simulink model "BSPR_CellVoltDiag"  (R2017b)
settings: Solver=FixedStepDiscrete  StartTime=0.0  StopTime=10.0  FixedStep=0.02  RelTol=1e-3  EnableMultiTasking=on
undefined symbols (not defined in the file): bin2dec, BSPR_bCellVoltAlrmDiag_C, BSPR_CellNplDetVoltThres_C, BSPR_cntCellAvlNum_C, BSPR_cntCellVltRngEnvtCsdr_CW, BSPR_cntCellVoltNplDiag_CW, BSPR_cntCellVoltRngDiag_CW, BSPR_cntModuAvlNum_C, BSPR_cntUCellNplErrThres_C, BSPR_cntUCellNplOkThres_C, BSPR_cntVoltCellMeanSwt_CW, BSPR_cofCurrFltCellRng_C, BSPR_iCellVoltRngCurrHi_C, BSPR_iCellVoltRngCurrLo_C, BSPR_iCurrHopFltDiff_C, BSPR_tBattTempCellVoltRngHi_C, BSPR_tBattTempCellVoltRngLo_C, BSPR_tEnvTCellVoltRngHi_C, BSPR_tEnvTCellVoltRnglo_C, BSPR_tiCellVoltAlrm_C, BSPR_tiCellVoltDiagTask_C, BSPR_tiCellVoltFault_C, BSPR_tiCellVoltFusf_C, BSPR_tiCellVoltWarn_C, BSPR_tiUCellNplErrThres_C, BSPR_tiUCellNplOkThres_C, BSPR_uCellVoltNplDiag_CUR, BSPR_uCellVoltNplDiag_CUR_X, BSPR_uCellVoltRng_CUR_X, BSPR_uCellVoltRng_CUR_Y, BSPR_uCellVoltRngHiFault_CUR, BSPR_uCellVoltRngHiFusf_CUR, BSPR_uCellVoltRngHiWarnAlrm_CUR, BSPR_uCellVoltRngLoFault_CUR, BSPR_uCellVoltRngLoFusf_CUR, BSPR_uCellVoltRngLoWarnAlrm_CUR
libraries: simulink x68, AIWAYS_Powertrain_BMS_lib x9
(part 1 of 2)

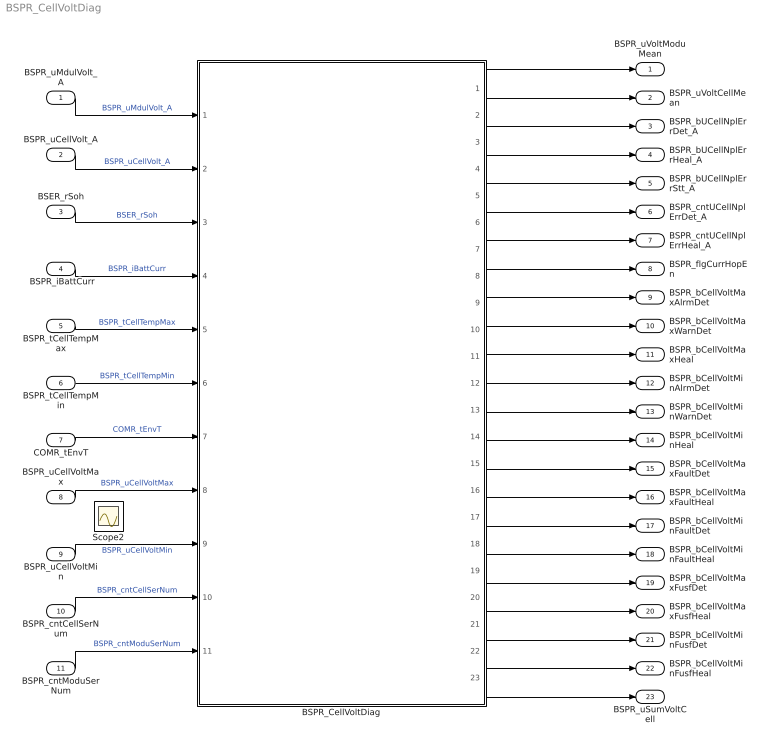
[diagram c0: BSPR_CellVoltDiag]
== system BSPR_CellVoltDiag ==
  BSPR_uMdulVolt_A : Inport
  BSPR_uCellVolt_A : Inport  Port=2
  BSER_rSoh : Inport  Port=3
  " BSPR_iBattCurr" : Inport  Port=4
  BSPR_tCellTempMax : Inport  Port=5
  BSPR_tCellTempMin : Inport  Port=6
  COMR_tEnvT : Inport  Port=7
  BSPR_uCellVoltMax : Inport  Port=8
  BSPR_uCellVoltMin : Inport  Port=9
  BSPR_cntCellSerNum : Inport  Port=10
  BSPR_cntModuSerNum : Inport  Port=11
  BSPR_CellVoltDiag : Subsystem
  BSPR_uVoltModuMean : Outport
  BSPR_uVoltCellMean : Outport  Port=2
  BSPR_bUCellNplErrDet_A : Outport  Port=3
  BSPR_bUCellNplErrHeal_A : Outport  Port=4
  BSPR_bUCellNplErrStt_A : Outport  Port=5
  BSPR_cntUCellNplErrDet_A : Outport  Port=6
  BSPR_cntUCellNplErrHeal_A : Outport  Port=7
  BSPR_flgCurrHopEn : Outport  Port=8
  BSPR_bCellVoltMaxAlrmDet : Outport  Port=9
  BSPR_bCellVoltMaxWarnDet : Outport  Port=10
  BSPR_bCellVoltMaxHeal : Outport  Port=11
  BSPR_bCellVoltMinAlrmDet : Outport  Port=12
  BSPR_bCellVoltMinWarnDet : Outport  Port=13
  BSPR_bCellVoltMinHeal : Outport  Port=14
  BSPR_bCellVoltMaxFaultDet : Outport  Port=15
  BSPR_bCellVoltMaxFaultHeal : Outport  Port=16
  BSPR_bCellVoltMinFaultDet : Outport  Port=17
  BSPR_bCellVoltMinFaultHeal : Outport  Port=18
  BSPR_bCellVoltMaxFusfDet : Outport  Port=19
  BSPR_bCellVoltMaxFusfHeal : Outport  Port=20
  BSPR_bCellVoltMinFusfDet : Outport  Port=21
  BSPR_bCellVoltMinFusfHeal : Outport  Port=22
  BSPR_uSumVoltCell : Outport  Port=23
  Scope2 : Scope
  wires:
  BSPR_uMdulVolt_A/1 -> BSPR_CellVoltDiag/1(BSPR_uMdulVolt_A)  "BSPR_uMdulVolt_A"
  BSPR_uCellVolt_A/1 -> BSPR_CellVoltDiag/2(BSPR_uCellVolt_A)  "BSPR_uCellVolt_A"
  BSER_rSoh/1 -> BSPR_CellVoltDiag/3(BSER_rSoh)  "BSER_rSoh"
  " BSPR_iBattCurr"/1 -> BSPR_CellVoltDiag/4(BSPR_iBattCurr)  "BSPR_iBattCurr"
  BSPR_tCellTempMax/1 -> BSPR_CellVoltDiag/5(BSPR_tCellTempMax)  "BSPR_tCellTempMax"
  BSPR_tCellTempMin/1 -> BSPR_CellVoltDiag/6(BSPR_tCellTempMin)  "BSPR_tCellTempMin"
  COMR_tEnvT/1 -> BSPR_CellVoltDiag/7(COMR_tEnvT)  "COMR_tEnvT"
  BSPR_uCellVoltMax/1 -> BSPR_CellVoltDiag/8(BSPR_uCellVoltMax)  "BSPR_uCellVoltMax"
  BSPR_uCellVoltMin/1 -> BSPR_CellVoltDiag/9(BSPR_uCellVoltMin)  "BSPR_uCellVoltMin"
  BSPR_CellVoltDiag/1(BSPR_uVoltModuMean) -> BSPR_uVoltModuMean/1
  BSPR_CellVoltDiag/2(BSPR_uVoltCellMean) -> BSPR_uVoltCellMean/1
  BSPR_CellVoltDiag/3(BSPR_bUCellNplErrDet_A) -> BSPR_bUCellNplErrDet_A/1
  BSPR_CellVoltDiag/4(BSPR_bUCellNplErrHeal_A) -> BSPR_bUCellNplErrHeal_A/1
  BSPR_CellVoltDiag/5(BSPR_bUCellNplErrStt_A) -> BSPR_bUCellNplErrStt_A/1
  BSPR_CellVoltDiag/6(BSPR_cntUCellNplErrDet_A) -> BSPR_cntUCellNplErrDet_A/1
  BSPR_CellVoltDiag/7(BSPR_cntUCellNplErrHeal_A) -> BSPR_cntUCellNplErrHeal_A/1
  BSPR_CellVoltDiag/8(BSPR_flgCurrHopEn) -> BSPR_flgCurrHopEn/1
  BSPR_CellVoltDiag/9(BSPR_bCellVoltMaxAlrmDet) -> BSPR_bCellVoltMaxAlrmDet/1
  BSPR_CellVoltDiag/10(BSPR_bCellVoltMaxWarnDet) -> BSPR_bCellVoltMaxWarnDet/1
  BSPR_CellVoltDiag/11(BSPR_bCellVoltMaxHeal) -> BSPR_bCellVoltMaxHeal/1
  BSPR_CellVoltDiag/12(BSPR_bCellVoltMinAlrmDet) -> BSPR_bCellVoltMinAlrmDet/1
  BSPR_CellVoltDiag/13(BSPR_bCellVoltMinWarnDet) -> BSPR_bCellVoltMinWarnDet/1
  BSPR_CellVoltDiag/14(BSPR_bCellVoltMinHeal) -> BSPR_bCellVoltMinHeal/1
  BSPR_CellVoltDiag/15(BSPR_bCellVoltMaxFaultDet) -> BSPR_bCellVoltMaxFaultDet/1
  BSPR_CellVoltDiag/16(BSPR_bCellVoltMaxFaultHeal) -> BSPR_bCellVoltMaxFaultHeal/1
  BSPR_CellVoltDiag/17(BSPR_bCellVoltMinFaultDet) -> BSPR_bCellVoltMinFaultDet/1
  BSPR_CellVoltDiag/18(BSPR_bCellVoltMinFaultHeal) -> BSPR_bCellVoltMinFaultHeal/1
  BSPR_CellVoltDiag/19(BSPR_bCellVoltMaxFusfDet) -> BSPR_bCellVoltMaxFusfDet/1
  BSPR_CellVoltDiag/20(BSPR_bCellVoltMaxFusfHeal) -> BSPR_bCellVoltMaxFusfHeal/1
  BSPR_CellVoltDiag/21(BSPR_bCellVoltMinFusfDet) -> BSPR_bCellVoltMinFusfDet/1
  BSPR_CellVoltDiag/22(BSPR_bCellVoltMinFusfHeal) -> BSPR_bCellVoltMinFusfHeal/1
  BSPR_cntCellSerNum/1 -> BSPR_CellVoltDiag/10(BSPR_cntCellSerNum)  "BSPR_cntCellSerNum"
  BSPR_CellVoltDiag/23(BSPR_uSumVoltCell) -> BSPR_uSumVoltCell/1
  BSPR_cntModuSerNum/1 -> BSPR_CellVoltDiag/11(BSPR_cntModuSerNum)  "BSPR_cntModuSerNum"

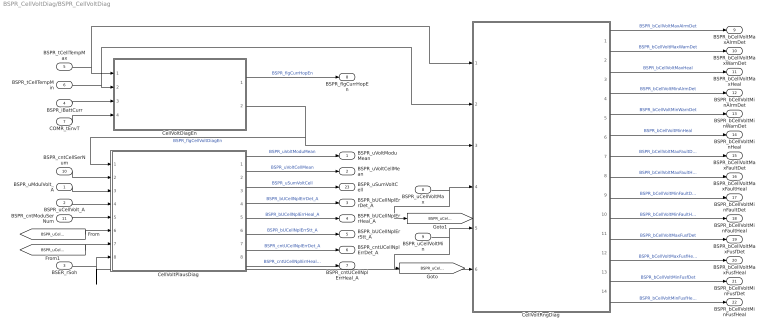
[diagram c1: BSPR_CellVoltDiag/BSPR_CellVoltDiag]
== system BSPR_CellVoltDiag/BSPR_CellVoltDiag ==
  BSPR_uMdulVolt_A : Inport
  BSPR_uCellVolt_A : Inport  Port=2
  BSER_rSoh : Inport  Port=3
  BSPR_iBattCurr : Inport  Port=4
  BSPR_tCellTempMax : Inport  Port=5
  BSPR_tCellTempMin : Inport  Port=6
  COMR_tEnvT : Inport  Port=7
  BSPR_uCellVoltMax : Inport  Port=8
  BSPR_uCellVoltMin : Inport  Port=9
  BSPR_cntCellSerNum : Inport  Port=10
  BSPR_cntModuSerNum : Inport  Port=11
  CellVoltDiagEn : Subsystem
  CellVoltPlausDiag : Subsystem
  CellVoltRngDiag : Subsystem
  BSPR_uVoltModuMean : Outport
  BSPR_uVoltCellMean : Outport  Port=2
  BSPR_bUCellNplErrDet_A : Outport  Port=3
  BSPR_bUCellNplErrHeal_A : Outport  Port=4
  BSPR_bUCellNplErrStt_A : Outport  Port=5
  BSPR_cntUCellNplErrDet_A : Outport  Port=6
  BSPR_cntUCellNplErrHeal_A : Outport  Port=7
  BSPR_flgCurrHopEn : Outport  Port=8
  BSPR_bCellVoltMaxAlrmDet : Outport  Port=9
  BSPR_bCellVoltMaxWarnDet : Outport  Port=10
  BSPR_bCellVoltMaxHeal : Outport  Port=11
  BSPR_bCellVoltMinAlrmDet : Outport  Port=12
  BSPR_bCellVoltMinWarnDet : Outport  Port=13
  BSPR_bCellVoltMinHeal : Outport  Port=14
  BSPR_bCellVoltMaxFaultDet : Outport  Port=15
  BSPR_bCellVoltMaxFaultHeal : Outport  Port=16
  BSPR_bCellVoltMinFaultDet : Outport  Port=17
  BSPR_bCellVoltMinFaultHeal : Outport  Port=18
  BSPR_bCellVoltMaxFusfDet : Outport  Port=19
  BSPR_bCellVoltMaxFusfHeal : Outport  Port=20
  BSPR_bCellVoltMinFusfDet : Outport  Port=21
  BSPR_bCellVoltMinFusfHeal : Outport  Port=22
  BSPR_uSumVoltCell : Outport  Port=23
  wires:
  BSPR_uCellVolt_A/1 -> CellVoltPlausDiag/4(BSPR_uCellVolt_A)
  BSPR_uMdulVolt_A/1 -> CellVoltPlausDiag/3(BSPR_uMdulVolt_A)
  BSER_rSoh/1 -> CellVoltPlausDiag/8(BSER_rSoh), CellVoltRngDiag/6(BSER_rSoh)
  CellVoltPlausDiag/1(BSPR_uVoltModuMean) -> BSPR_uVoltModuMean/1  "BSPR_uVoltModuMean"
  CellVoltPlausDiag/5(BSPR_bUCellNplErrHeal_A) -> BSPR_bUCellNplErrHeal_A/1  "BSPR_bUCellNplErrHeal_A"
  CellVoltPlausDiag/4(BSPR_bUCellNplErrDet_A) -> BSPR_bUCellNplErrDet_A/1  "BSPR_bUCellNplErrDet_A"
  CellVoltPlausDiag/2(BSPR_uVoltCellMean) -> BSPR_uVoltCellMean/1  "BSPR_uVoltCellMean"
  CellVoltPlausDiag/6(BSPR_bUCellNplErrStt_A) -> BSPR_bUCellNplErrStt_A/1  "BSPR_bUCellNplErrStt_A"
  CellVoltPlausDiag/7(BSPR_cntUCellNplErrDet_A) -> BSPR_cntUCellNplErrDet_A/1  "BSPR_cntUCellNplErrDet_A"
  CellVoltPlausDiag/8(BSPR_cntUCellNplErrHeal_A) -> BSPR_cntUCellNplErrHeal_A/1  "BSPR_cntUCellNplErrHeal_A"
  CellVoltDiagEn/1(BSPR_flgCurrHopEn) -> BSPR_flgCurrHopEn/1  "BSPR_flgCurrHopEn"
  BSPR_tCellTempMax/1 -> CellVoltDiagEn/1(BSPR_tCellTempMax), CellVoltRngDiag/1(BSPR_tCellTempMax)
  BSPR_tCellTempMin/1 -> CellVoltRngDiag/2(BSPR_tCellTempMin), CellVoltDiagEn/2(BSPR_tCellTempMin)
  BSPR_iBattCurr/1 -> CellVoltDiagEn/3(BSPR_iBattCurr)
  COMR_tEnvT/1 -> CellVoltDiagEn/4(COMR_tEnvT)
  CellVoltDiagEn/2(BSPR_flgCellVoltDiagEn) -> CellVoltPlausDiag/1(BSPR_flgCellVoltDiagEn), CellVoltRngDiag/3(BSPR_flgCellVoltDiagEn)  "BSPR_flgCellVoltDiagEn"
  CellVoltRngDiag/1(BSPR_bCellVoltMaxAlrmDet) -> BSPR_bCellVoltMaxAlrmDet/1  "BSPR_bCellVoltMaxAlrmDet"
  CellVoltRngDiag/2(BSPR_bCellVoltMaxWarnDet) -> BSPR_bCellVoltMaxWarnDet/1  "BSPR_bCellVoltMaxWarnDet"
  CellVoltRngDiag/3(BSPR_bCellVoltMaxHeal) -> BSPR_bCellVoltMaxHeal/1  "BSPR_bCellVoltMaxHeal"
  CellVoltRngDiag/4(BSPR_bCellVoltMinAlrmDet) -> BSPR_bCellVoltMinAlrmDet/1  "BSPR_bCellVoltMinAlrmDet"
  CellVoltRngDiag/5(BSPR_bCellVoltMinWarnDet) -> BSPR_bCellVoltMinWarnDet/1  "BSPR_bCellVoltMinWarnDet"
  CellVoltRngDiag/7(BSPR_bCellVoltMaxFaultDet) -> BSPR_bCellVoltMaxFaultDet/1  "BSPR_bCellVoltMaxFaultDet"
  CellVoltRngDiag/9(BSPR_bCellVoltMinFaultDet) -> BSPR_bCellVoltMinFaultDet/1  "BSPR_bCellVoltMinFaultDet"
  CellVoltRngDiag/10(BSPR_bCellVoltMinFaultHeal) -> BSPR_bCellVoltMinFaultHeal/1  "BSPR_bCellVoltMinFaultHeal"
  CellVoltRngDiag/11(BSPR_bCellVoltMaxFusfDet) -> BSPR_bCellVoltMaxFusfDet/1  "BSPR_bCellVoltMaxFusfDet"
  CellVoltRngDiag/13(BSPR_bCellVoltMinFusfDet) -> BSPR_bCellVoltMinFusfDet/1  "BSPR_bCellVoltMinFusfDet"
  CellVoltRngDiag/14(BSPR_bCellVoltMinFusfHeal) -> BSPR_bCellVoltMinFusfHeal/1  "BSPR_bCellVoltMinFusfHeal"
  BSPR_uCellVoltMax/1 -> [BSPR_uCellVoltMax], CellVoltRngDiag/4(BSPR_uCellVoltMax)
  BSPR_uCellVoltMin/1 -> [BSPR_uCellVoltMin], CellVoltRngDiag/5(BSPR_uCellVoltMin)
  CellVoltRngDiag/6(BSPR_bCellVoltMinHeal) -> BSPR_bCellVoltMinHeal/1  "BSPR_bCellVoltMinHeal"
  CellVoltRngDiag/8(BSPR_bCellVoltMaxFaultHeal) -> BSPR_bCellVoltMaxFaultHeal/1  "BSPR_bCellVoltMaxFaultHeal"
  CellVoltRngDiag/12(BSPR_bCellVoltMaxFusfHeal) -> BSPR_bCellVoltMaxFusfHeal/1  "BSPR_bCellVoltMaxFusfHeal"
  BSPR_cntCellSerNum/1 -> CellVoltPlausDiag/2(BSPR_cntCellSerNum)
  CellVoltPlausDiag/3(BSPR_uSumVoltCell) -> BSPR_uSumVoltCell/1  "BSPR_uSumVoltCell"
  BSPR_cntModuSerNum/1 -> CellVoltPlausDiag/5(BSPR_cntModuSerNum)
  [BSPR_uCellVoltMin] -> CellVoltPlausDiag/6(BSPR_uCellVoltMin)
  [BSPR_uCellVoltMax] -> CellVoltPlausDiag/7(BSPR_uCellVoltMax)

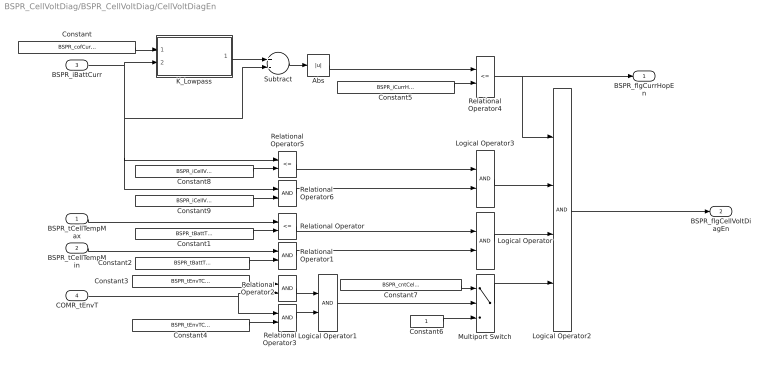
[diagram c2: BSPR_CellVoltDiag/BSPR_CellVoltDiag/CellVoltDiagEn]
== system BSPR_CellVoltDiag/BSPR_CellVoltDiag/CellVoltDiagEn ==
  BSPR_tCellTempMax : Inport
  BSPR_tCellTempMin : Inport  Port=2
  BSPR_iBattCurr : Inport  Port=3
  COMR_tEnvT : Inport  Port=4
  Abs : Abs
  Constant : Constant  Value=BSPR_cofCurrFltCellRng_C
  Constant1 : Constant  Value=BSPR_tBattTempCellVoltRngHi_C
  Constant2 : Constant  Value=BSPR_tBattTempCellVoltRngLo_C
  Constant3 : Constant  Value=BSPR_tEnvTCellVoltRngHi_C
  Constant4 : Constant  Value=BSPR_tEnvTCellVoltRnglo_C
  Constant5 : Constant  Value=BSPR_iCurrHopFltDiff_C
  Constant6 : Constant
  Constant7 : Constant  Value=BSPR_cntCellVltRngEnvtCsdr_CW  OutMin=[0]  OutMax=[1]
  Constant8 : Constant  Value=BSPR_iCellVoltRngCurrHi_C
  Constant9 : Constant  Value=BSPR_iCellVoltRngCurrLo_C
  K_Lowpass : Subsystem  TreatAsAtomicUnit=on  RTWFcnName=K_Lowpass  RTWFileName=SrvLib
  Logical Operator : Logic  AllPortsSameDT=off  OutDataTypeStr=boolean
  Logical Operator1 : Logic  AllPortsSameDT=off  OutDataTypeStr=boolean
  Logical Operator2 : Logic  Inputs=4  AllPortsSameDT=off  OutDataTypeStr=boolean
  Logical Operator3 : Logic  AllPortsSameDT=off  OutDataTypeStr=boolean
  Multiport Switch : MultiPortSwitch  DataPortOrder=Zero-based contiguous  Inputs=2
  Relational Operator : RelationalOperator  Operator=<=  OutDataTypeStr=boolean  RndMeth=Simplest
  Relational Operator{1..3,6} (4 alike) : RelationalOperator  OutDataTypeStr=boolean  RndMeth=Simplest
  Relational Operator4 : RelationalOperator  Operator=<=  OutDataTypeStr=boolean  RndMeth=Simplest
  Relational Operator5 : RelationalOperator  Operator=<=  OutDataTypeStr=boolean  RndMeth=Simplest
  Subtract : Sum  Inputs=+-
  BSPR_flgCurrHopEn : Outport
  BSPR_flgCellVoltDiagEn : Outport  Port=2
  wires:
  K_Lowpass/1(y) -> Subtract/1
  Subtract/1 -> Abs/1
  Abs/1 -> Relational Operator4/1
  Constant6/1 -> Multiport Switch/3
  Multiport Switch/1 -> Logical Operator2/4
  Constant3/1 -> Relational Operator2/1
  Constant4/1 -> Relational Operator3/2
  COMR_tEnvT/1 -> Relational Operator3/1, Relational Operator2/2
  Constant1/1 -> Relational Operator/2
  Constant2/1 -> Relational Operator1/2
  BSPR_tCellTempMin/1 -> Relational Operator1/1
  BSPR_iBattCurr/1 -> K_Lowpass/2(u), Relational Operator6/1, Relational Operator5/1, Subtract/2
  BSPR_tCellTempMax/1 -> Relational Operator/1
  Relational Operator1/1 -> Logical Operator/2
  Relational Operator3/1 -> Logical Operator1/2
  Relational Operator2/1 -> Logical Operator1/1
  Constant7/1 -> Multiport Switch/1
  Relational Operator/1 -> Logical Operator/1
  Logical Operator1/1 -> Multiport Switch/2
  Relational Operator4/1 -> BSPR_flgCurrHopEn/1, Logical Operator2/1
  Constant5/1 -> Relational Operator4/2
  Logical Operator/1 -> Logical Operator2/3
  Logical Operator2/1 -> BSPR_flgCellVoltDiagEn/1
  Constant/1 -> K_Lowpass/1(k)
  Constant9/1 -> Relational Operator6/2
  Constant8/1 -> Relational Operator5/2
  Relational Operator5/1 -> Logical Operator3/1
  Relational Operator6/1 -> Logical Operator3/2
  Logical Operator3/1 -> Logical Operator2/2

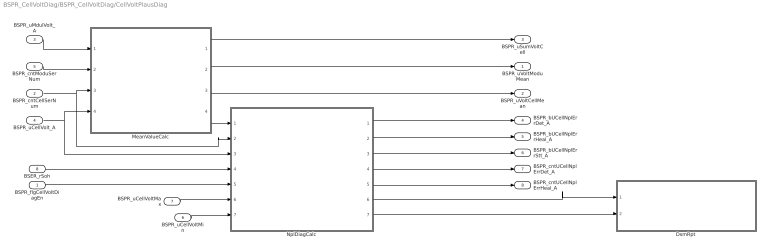
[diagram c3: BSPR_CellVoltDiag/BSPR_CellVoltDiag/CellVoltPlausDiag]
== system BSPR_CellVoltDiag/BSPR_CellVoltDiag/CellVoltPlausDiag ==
  BSPR_flgCellVoltDiagEn : Inport
  BSPR_cntCellSerNum : Inport  Port=2
  BSPR_uMdulVolt_A : Inport  Port=3
  BSPR_uCellVolt_A : Inport  Port=4
  BSPR_cntModuSerNum : Inport  Port=5
  BSPR_uCellVoltMin : Inport  Port=6
  BSPR_uCellVoltMax : Inport  Port=7
  BSER_rSoh : Inport  Port=8
  DsmRpt : Subsystem
  MeanValueCalc : Subsystem
  NplDiagCalc : Subsystem
  BSPR_uVoltModuMean : Outport
  BSPR_uVoltCellMean : Outport  Port=2
  BSPR_uSumVoltCell : Outport  Port=3
  BSPR_bUCellNplErrDet_A : Outport  Port=4  InitialOutput=[0]
  BSPR_bUCellNplErrHeal_A : Outport  Port=5  InitialOutput=[0]
  BSPR_bUCellNplErrStt_A : Outport  Port=6  InitialOutput=[0]
  BSPR_cntUCellNplErrDet_A : Outport  Port=7  InitialOutput=[0]
  BSPR_cntUCellNplErrHeal_A : Outport  Port=8  InitialOutput=[0]
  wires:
  BSPR_uMdulVolt_A/1 -> MeanValueCalc/1(BSPR_uMdulVolt_A)
  MeanValueCalc/2(BSPR_uVoltModuMean) -> BSPR_uVoltModuMean/1
  MeanValueCalc/4(BSPR_uCellVoltMeanCoord) -> NplDiagCalc/1(BSPR_uCellVoltMeanCoord)
  NplDiagCalc/2(BSPR_bUCellNplErrHeal_A) -> BSPR_bUCellNplErrHeal_A/1
  NplDiagCalc/1(BSPR_bUCellNplErrDet_A) -> BSPR_bUCellNplErrDet_A/1
  BSER_rSoh/1 -> NplDiagCalc/4(BSER_rSoh)
  MeanValueCalc/3(BSPR_uVoltCellMean) -> BSPR_uVoltCellMean/1
  NplDiagCalc/3(BSPR_bUCellNplErrStt_A) -> BSPR_bUCellNplErrStt_A/1
  NplDiagCalc/4(BSPR_cntUCellNplErrDet_A) -> BSPR_cntUCellNplErrDet_A/1
  NplDiagCalc/5(BSPR_cntUCellNplErrHeal_A) -> BSPR_cntUCellNplErrHeal_A/1
  BSPR_uCellVolt_A/1 -> MeanValueCalc/4(BSPR_uCellVolt_A), NplDiagCalc/3(BSPR_uCellVolt_A)
  BSPR_flgCellVoltDiagEn/1 -> NplDiagCalc/5(BSPR_flgCellVoltDiagEn)
  MeanValueCalc/1(BSPR_uSumVoltCell) -> BSPR_uSumVoltCell/1
  BSPR_cntCellSerNum/1 -> MeanValueCalc/3(BSPR_cntCellSerNum), NplDiagCalc/2(BSPR_cntCellSerNum)
  BSPR_cntModuSerNum/1 -> MeanValueCalc/2(BSPR_cntModuSerNum)
  BSPR_uCellVoltMin/1 -> NplDiagCalc/7(BSPR_uCellVoltMin)
  BSPR_uCellVoltMax/1 -> NplDiagCalc/6(BSPR_uCellVoltMax)
  NplDiagCalc/6(BSPR_bUCellNplErrDet_flg) -> DsmRpt/1(BSPR_bUCellNplErrDet_flg)
  NplDiagCalc/7(BSPR_bUCellNplErrHeal_flg) -> DsmRpt/2(BSPR_bUCellNplErrHeal_flg)

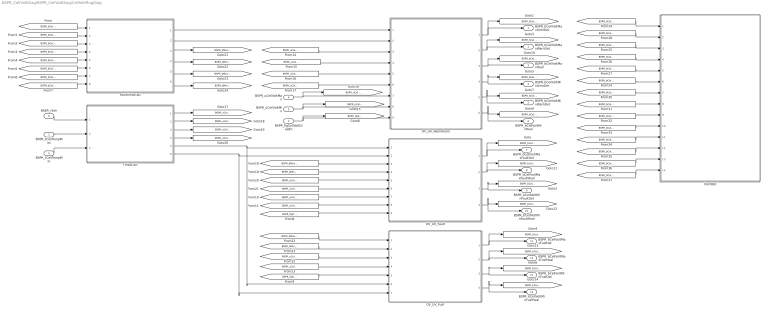
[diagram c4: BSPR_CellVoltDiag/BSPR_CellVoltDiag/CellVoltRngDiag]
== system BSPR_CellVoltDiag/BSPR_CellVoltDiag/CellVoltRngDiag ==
  BSPR_tCellTempMax : Inport
  BSPR_tCellTempMin : Inport  Port=2
  BSPR_flgCellVoltDiagEn : Inport  Port=3
  BSPR_uCellVoltMax : Inport  Port=4
  BSPR_uCellVoltMin : Inport  Port=5
  BSER_rSoh : Inport  Port=6
  DsmRpt : Subsystem
  FaultInhibCalc : Subsystem
  OV_UV_Fault : Subsystem
  OV_UV_Fusf : Subsystem
  OV_UV_WarnAlarm : Subsystem
  ThresCalc : Subsystem
  BSPR_bCellVoltMaxAlrmDet : Outport  InitialOutput=[0]
  BSPR_bCellVoltMaxWarnDet : Outport  Port=2  InitialOutput=[0]
  BSPR_bCellVoltMaxHeal : Outport  Port=3  InitialOutput=[0]
  BSPR_bCellVoltMinAlrmDet : Outport  Port=4  InitialOutput=[0]
  BSPR_bCellVoltMinWarnDet : Outport  Port=5  InitialOutput=[0]
  BSPR_bCellVoltMinHeal : Outport  Port=6  InitialOutput=[0]
  BSPR_bCellVoltMaxFaultDet : Outport  Port=7  InitialOutput=[0]
  BSPR_bCellVoltMaxFaultHeal : Outport  Port=8  InitialOutput=[0]
  BSPR_bCellVoltMinFaultDet : Outport  Port=9  InitialOutput=[0]
  BSPR_bCellVoltMinFaultHeal : Outport  Port=10  InitialOutput=[0]
  BSPR_bCellVoltMaxFusfDet : Outport  Port=11  InitialOutput=[0]
  BSPR_bCellVoltMaxFusfHeal : Outport  Port=12  InitialOutput=[0]
  BSPR_bCellVoltMinFusfDet : Outport  Port=13  InitialOutput=[0]
  BSPR_bCellVoltMinFusfHeal : Outport  Port=14  InitialOutput=[0]
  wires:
  OV_UV_WarnAlarm/6(BSPR_bCellVoltMinHeal) -> BSPR_bCellVoltMinHeal/1, [BSPR_bCellVoltMinHeal]
  OV_UV_WarnAlarm/5(BSPR_bCellVoltMinWarnDet) -> BSPR_bCellVoltMinWarnDet/1, [BSPR_bCellVoltMinWarnDet]
  OV_UV_WarnAlarm/4(BSPR_bCellVoltMinAlrmDet) -> BSPR_bCellVoltMinAlrmDet/1, [BSPR_bCellVoltMinAlrmDet]
  OV_UV_WarnAlarm/3(BSPR_bCellVoltMaxHeal) -> BSPR_bCellVoltMaxHeal/1, [BSPR_bCellVoltMaxHeal]
  OV_UV_WarnAlarm/2(BSPR_bCellVoltMaxWarnDet) -> BSPR_bCellVoltMaxWarnDet/1, [BSPR_bCellVoltMaxWarnDet]
  OV_UV_WarnAlarm/1(BSPR_bCellVoltMaxAlrmDet) -> BSPR_bCellVoltMaxAlrmDet/1, [BSPR_bCellVoltMaxAlrmDet]
  BSER_rSoh/1 -> ThresCalc/1(BSER_rSoh)
  OV_UV_Fault/1(BSPR_bCellVoltMaxFaultDet) -> [BSPR_bCellVoltMaxFaultDet], BSPR_bCellVoltMaxFaultDet/1
  OV_UV_Fault/3(BSPR_bCellVoltMinFaultDet) -> [BSPR_bCellVoltMinFaultDet], BSPR_bCellVoltMinFaultDet/1
  OV_UV_Fault/4(BSPR_bCellVoltMinFaultHeal) -> [BSPR_bCellVoltMinFaultHeal], BSPR_bCellVoltMinFaultHeal/1
  ThresCalc/5(BSPR_uCellVoltRngHiFusf) -> OV_UV_Fault/1(BSPR_uCellVoltRngHiFusf), OV_UV_Fusf/6(BSPR_uCellVoltRngHiFusf)
  ThresCalc/6(BSPR_uCellVoltRngLoFusf) -> OV_UV_Fault/2(BSPR_uCellVoltRngLoFusf), OV_UV_Fusf/7(BSPR_uCellVoltRngLoFusf)
  BSPR_uCellVoltMax/1 -> [BSPR_uCellVoltMax], OV_UV_WarnAlarm/7(BSPR_uCellVoltMax)
  BSPR_uCellVoltMin/1 -> [BSPR_uCellVoltMin], OV_UV_WarnAlarm/8(BSPR_uCellVoltMin)
  OV_UV_Fusf/1(BSPR_bCellVoltMaxFusfDet) -> BSPR_bCellVoltMaxFusfDet/1, [BSPR_bCellVoltMaxFusfDet]
  OV_UV_Fusf/2(BSPR_bCellVoltMaxFusfHeal) -> [BSPR_bCellVoltMaxFusfHeal], BSPR_bCellVoltMaxFusfHeal/1
  OV_UV_Fusf/3(BSPR_bCellVoltMinFusfDet) -> [BSPR_bCellVoltMinFusfDet], BSPR_bCellVoltMinFusfDet/1
  OV_UV_Fusf/4(BSPR_bCellVoltMinFusfHeal) -> [BSPR_bCellVoltMinFusfHeal], BSPR_bCellVoltMinFusfHeal/1
  [BSPR_bCellVoltMaxAlrmDet] -> FaultInhibCalc/1(BSPR_bCellVoltMaxAlrmDet)
  [BSPR_bCellVoltMaxWarnDet] -> FaultInhibCalc/2(BSPR_bCellVoltMaxWarnDet)
  [BSPR_bCellVoltMinAlrmDet] -> FaultInhibCalc/3(BSPR_bCellVoltMinAlrmDet)
  [BSPR_bCellVoltMinWarnDet] -> FaultInhibCalc/4(BSPR_bCellVoltMinWarnDet)
  [BSPR_bCellVoltMinFusfDet] -> FaultInhibCalc/8(BSPR_bCellVoltMinFusfDet)
  [BSPR_bCellVoltMaxFaultDet] -> FaultInhibCalc/5(BSPR_bCellVoltMaxFaultDet)
  [BSPR_bCellVoltMinFaultDet] -> FaultInhibCalc/6(BSPR_bCellVoltMinFaultDet)
  [BSPR_bCellVoltMaxFusfDet] -> FaultInhibCalc/7(BSPR_bCellVoltMaxFusfDet)
  FaultInhibCalc/1(BSPR_bMaxAlrmWarnInhib) -> OV_UV_WarnAlarm/1(BSPR_bMaxAlrmWarnInhib)
  FaultInhibCalc/2(BSPR_bMinAlrmWarnInhib) -> OV_UV_WarnAlarm/2(BSPR_bMinAlrmWarnInhib)
  BSPR_tCellTempMin/1 -> ThresCalc/3(BSPR_tCellTempMin)
  BSPR_tCellTempMax/1 -> ThresCalc/2(BSPR_tCellTempMax)
  BSPR_flgCellVoltDiagEn/1 -> OV_UV_WarnAlarm/9(BSPR_flgCellVoltDiagEn), [BSPR_flgCellVoltDiagEn]
  [BSPR_flgCellVoltDiagEn] -> OV_UV_Fault/9(BSPR_flgCellVoltDiagEn)
  [BSPR_flgCellVoltDiagEn] -> OV_UV_Fusf/5(BSPR_flgCellVoltDiagEn)
  OV_UV_Fault/2(BSPR_bCellVoltMaxFaultHeal) -> [BSPR_bCellVoltMaxFaultHeal], BSPR_bCellVoltMaxFaultHeal/1
  [BSPR_uCellVoltMin] -> OV_UV_Fault/8(BSPR_uCellVoltMin)
  [BSPR_uCellVoltMax] -> OV_UV_Fault/7(BSPR_uCellVoltMax)
  [BSPR_uCellVoltMax] -> OV_UV_Fusf/3(BSPR_uCellVoltMax)
  [BSPR_uCellVoltMin] -> OV_UV_Fusf/4(BSPR_uCellVoltMin)
  ThresCalc/1(BSPR_uCellVoltRngHiWarnAlrm) -> [BSPR_uCellVoltRngHiWarnAlrm]
  ThresCalc/2(BSPR_uCellVoltRngLoWarnAlrm) -> [BSPR_uCellVoltRngLoWarnAlrm]
  ThresCalc/3(BSPR_uCellVoltRngHiFault) -> [BSPR_uCellVoltRngHiFault]
  ThresCalc/4(BSPR_uCellVoltRngLoFault) -> [BSPR_uCellVoltRngLoFault]
  [BSPR_uCellVoltRngHiWarnAlrm] -> OV_UV_WarnAlarm/3(BSPR_uCellVoltRngHiWarnAlrm)
  [BSPR_uCellVoltRngLoWarnAlrm] -> OV_UV_WarnAlarm/4(BSPR_uCellVoltRngLoWarnAlrm)
  [BSPR_uCellVoltRngHiFault] -> OV_UV_WarnAlarm/5(BSPR_uCellVoltRngHiFault)
  [BSPR_uCellVoltRngLoFault] -> OV_UV_WarnAlarm/6(BSPR_uCellVoltRngLoFault)
  FaultInhibCalc/3(BSPR_bMaxFaultInhib) -> [BSPR_bMaxFaultInhib]
  FaultInhibCalc/4(BSPR_bMinFaultInhib) -> [BSPR_bMinFaultInhib]
  FaultInhibCalc/5(BSPR_bMaxFusfInhib) -> [BSPR_bMaxFusfInhib]
  FaultInhibCalc/6(BSPR_bMinFusfInhib) -> [BSPR_bMinFusfInhib]
  [BSPR_bMaxFaultInhib] -> OV_UV_Fault/3(BSPR_bMaxFaultInhib)
  [BSPR_bMinFaultInhib] -> OV_UV_Fault/4(BSPR_bMinFaultInhib)
  [BSPR_uCellVoltRngLoFault] -> OV_UV_Fault/6(BSPR_uCellVoltRngLoFault)
  [BSPR_uCellVoltRngHiFault] -> OV_UV_Fault/5(BSPR_uCellVoltRngHiFault)
  [BSPR_bMaxFusfInhib] -> OV_UV_Fusf/1(BSPR_bMaxFusfInhib)
  [BSPR_bMinFusfInhib] -> OV_UV_Fusf/2(BSPR_bMinFusfInhib)
  [BSPR_bCellVoltMaxAlrmDet] -> DsmRpt/1(BSPR_bCellVoltMaxAlrmDet)
  [BSPR_bCellVoltMaxWarnDet] -> DsmRpt/2(BSPR_bCellVoltMaxWarnDet)
  [BSPR_bCellVoltMaxHeal] -> DsmRpt/3(BSPR_bCellVoltMaxHeal)
  [BSPR_bCellVoltMinAlrmDet] -> DsmRpt/4(BSPR_bCellVoltMinAlrmDet)
  [BSPR_bCellVoltMinWarnDet] -> DsmRpt/5(BSPR_bCellVoltMinWarnDet)
  [BSPR_bCellVoltMinHeal] -> DsmRpt/6(BSPR_bCellVoltMinHeal)
  [BSPR_bCellVoltMaxFaultDet] -> DsmRpt/7(BSPR_bCellVoltMaxFaultDet)
  [BSPR_bCellVoltMaxFaultHeal] -> DsmRpt/8(BSPR_bCellVoltMaxFaultHeal)
  [BSPR_bCellVoltMinFaultDet] -> DsmRpt/9(BSPR_bCellVoltMinFaultDet)
  [BSPR_bCellVoltMinFaultHeal] -> DsmRpt/10(BSPR_bCellVoltMinFaultHeal)
  [BSPR_bCellVoltMaxFusfDet] -> DsmRpt/11(BSPR_bCellVoltMaxFusfDet)
  [BSPR_bCellVoltMaxFusfHeal] -> DsmRpt/12(BSPR_bCellVoltMaxFusfHeal)
  [BSPR_bCellVoltMinFusfHeal] -> DsmRpt/14(BSPR_bCellVoltMinFusfHeal)
  [BSPR_bCellVoltMinFusfDet] -> DsmRpt/13(BSPR_bCellVoltMinFusfDet)

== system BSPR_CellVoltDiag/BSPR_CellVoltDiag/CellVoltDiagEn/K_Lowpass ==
  k : Inport
  u : Inport  Port=2
  Add : Sum
  Constant2 : Constant  Value=0
  Delay : Delay  DelayLength=1  InitialCondition=1
  Product : Product
  Subtract : Sum  Inputs=+-
  Switch1 : Switch  Criteria=u2 > Threshold
  Unit Delay : UnitDelay  SampleTime=-1
  y : Outport
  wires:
  u/1 -> Subtract/1, Switch1/1
  Switch1/1 -> Unit Delay/1, y/1
  Delay/1 -> Switch1/2
  Add/1 -> Switch1/3
  Subtract/1 -> Product/2
  Unit Delay/1 -> Add/2, Subtract/2
  Constant2/1 -> Delay/1
  Product/1 -> Add/1
  k/1 -> Product/1

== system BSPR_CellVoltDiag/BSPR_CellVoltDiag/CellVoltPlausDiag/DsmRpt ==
  BSPR_bUCellNplErrDet_flg : Inport
  BSPR_bUCellNplErrHeal_flg : Inport  Port=2
  Bitwise Operator : simulink/Logic and Bit Operations/Bitwise Operator  logicop=AND  UseBitMask=on  BitMask=bin2dec('00000001')  BitMaskRealWorld=Stored Integer
  Compare To Constant4 : simulink/Logic and Bit Operations/Compare To Constant  relop===  const=1  OutDataTypeStr=boolean
  Constant : Constant  Value=BSPR_cntCellVoltNplDiag_CW
  Constant1 : Constant  OutDataTypeStr=boolean
  Constant2 : Constant  Value=0  OutDataTypeStr=boolean
  DSM_ReportCheck : Subsystem  TreatAsAtomicUnit=on  RTWFcnName=DSM_ReportCheck  RTWFileName=SrvLib
  Data Store Read : DataStoreRead  DataStoreName=DFC_CellVoltNpl
  Data Store Write : DataStoreWrite  DataStoreName=DFC_CellVoltNpl
  Switch : Switch  Criteria=u2 > Threshold
  Switch1 : Switch  Criteria=u2 > Threshold
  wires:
  DSM_ReportCheck/1(Dfc_id) -> Data Store Write/1
  BSPR_bUCellNplErrDet_flg/1 -> Switch/1
  BSPR_bUCellNplErrHeal_flg/1 -> Switch1/1
  Data Store Read/1 -> DSM_ReportCheck/1(Dfc_id_nv)
  Constant/1 -> Bitwise Operator/1
  Bitwise Operator/1 -> Compare To Constant4/1
  Constant2/1 -> Switch/3
  Constant1/1 -> Switch1/3
  Switch/1 -> DSM_ReportCheck/2(Err)
  Switch1/1 -> DSM_ReportCheck/3(Heal)
  Compare To Constant4/1 -> Switch1/2, Switch/2

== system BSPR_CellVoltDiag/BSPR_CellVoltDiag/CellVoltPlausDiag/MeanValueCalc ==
  BSPR_uMdulVolt_A : Inport
  BSPR_cntModuSerNum : Inport  Port=2
  BSPR_cntCellSerNum : Inport  Port=3
  BSPR_uCellVolt_A : Inport  Port=4
  CellVolt_SglProc : Subsystem
  MeanValueCalcCell : Subsystem
  MeanValueCalcModu : Subsystem
  MeanValueChoose : Subsystem
  ModuVolt_SglProc : Subsystem
  BSPR_uSumVoltCell : Outport
  BSPR_uVoltModuMean : Outport  Port=2
  BSPR_uVoltCellMean : Outport  Port=3
  BSPR_uCellVoltMeanCoord : Outport  Port=4
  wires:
  BSPR_uCellVolt_A/1 -> CellVolt_SglProc/1(BSPR_uCellVolt_A)
  CellVolt_SglProc/1(BSPR_uSumVoltCellTmp) -> MeanValueCalcCell/1(BSPR_uSumVoltCellTmp)
  CellVolt_SglProc/2(BSPR_uSumExtmVoltCell) -> MeanValueCalcCell/2(BSPR_uSumExtmVoltCell)
  BSPR_cntCellSerNum/1 -> CellVolt_SglProc/2(BSPR_cntCellSerNum), MeanValueChoose/3(BSPR_cntCellSerNum), MeanValueCalcCell/3(BSPR_cntCellSerNum)
  BSPR_cntModuSerNum/1 -> MeanValueCalcModu/3(BSPR_cntModuSerNum), ModuVolt_SglProc/2(BSPR_cntModuSerNum)
  ModuVolt_SglProc/2(BSPR_uSumExtmVoltModu) -> MeanValueCalcModu/2(BSPR_uSumExtmVoltModu)
  ModuVolt_SglProc/1(BSPR_uSumVoltModuTmp) -> MeanValueCalcModu/1(BSPR_uSumVoltModuTmp)
  BSPR_uMdulVolt_A/1 -> ModuVolt_SglProc/1(BSPR_uMdulVolt_A)
  MeanValueChoose/1(BSPR_uCellVoltMeanCoord) -> BSPR_uCellVoltMeanCoord/1  "BSPR_uCellVoltMeanCoord"
  MeanValueCalcModu/1(BSPR_uVoltModuMean) -> MeanValueChoose/1(BSPR_uVoltModuMean), BSPR_uVoltModuMean/1
  MeanValueCalcCell/1(BSPR_uVoltCellMean) -> MeanValueChoose/2(BSPR_uVoltCellMean), BSPR_uVoltCellMean/1
  MeanValueChoose/2(BSPR_uSumVoltCell) -> BSPR_uSumVoltCell/1

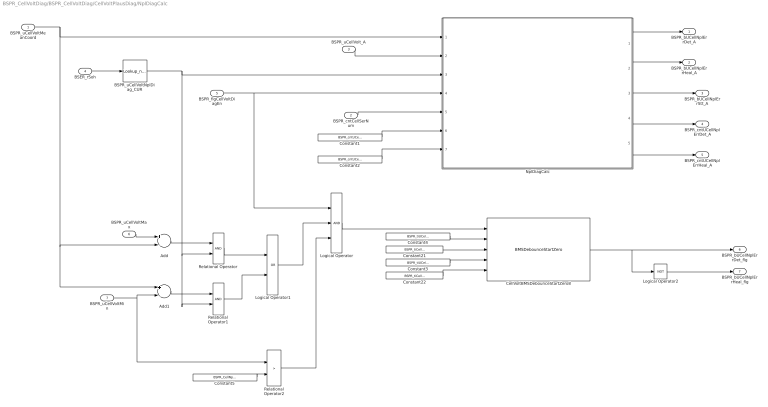
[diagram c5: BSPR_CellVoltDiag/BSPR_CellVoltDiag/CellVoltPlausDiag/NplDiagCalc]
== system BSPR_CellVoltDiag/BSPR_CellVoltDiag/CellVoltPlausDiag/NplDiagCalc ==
  BSPR_uCellVoltMeanCoord : Inport
  BSPR_cntCellSerNum : Inport  Port=2
  BSPR_uCellVolt_A : Inport  Port=3
  BSER_rSoh : Inport  Port=4
  BSPR_flgCellVoltDiagEn : Inport  Port=5
  BSPR_uCellVoltMax : Inport  Port=6
  BSPR_uCellVoltMin : Inport  Port=7
  Add : Sum  Inputs=+-
  Add1 : Sum  Inputs=+-
  BSPR_uCellVoltNplDiag_CUR : Lookup_n-D  NumberOfTableDimensions=1  LookupTableObject=qdwq  BreakpointsForDimension1=BSPR_uCellVoltNplDiag_CUR_X  Table=BSPR_uCellVoltNplDiag_CUR  InternalRulePriority=Speed  OutMin=[0]  OutMax=[100]  RndMeth=Simplest  SaturateOnIntegerOverflow=on
  CellVoltBMSDebounceStartZero8 : AIWAYS_Powertrain_BMS_lib/Debounce & Delay/BMSDebounceStartZero
  Constant1 : Constant  Value=BSPR_cntUCellNplOkThres_C
  Constant2 : Constant  Value=BSPR_cntUCellNplErrThres_C
  Constant21 : Constant  Value=BSPR_tiCellVoltDiagTask_C
  Constant22 : Constant  Value=BSPR_tiCellVoltDiagTask_C
  Constant3 : Constant  Value=BSPR_tiUCellNplOkThres_C  VectorParams1D=off
  Constant4 : Constant  Value=BSPR_tiUCellNplErrThres_C
  Constant5 : Constant  Value=BSPR_CellNplDetVoltThres_C
  Logical Operator : Logic  Inputs=3  AllPortsSameDT=off  OutDataTypeStr=boolean
  Logical Operator1 : Logic  Operator=OR  AllPortsSameDT=off  OutDataTypeStr=boolean
  Logical Operator2 : Logic  Operator=NOT  AllPortsSameDT=off  OutDataTypeStr=boolean
  NplDiagCalc : Stateflow chart  TreatAsAtomicUnit=on
  Relational Operator : RelationalOperator  OutDataTypeStr=boolean  RndMeth=Simplest
  Relational Operator1 : RelationalOperator  OutDataTypeStr=boolean  RndMeth=Simplest
  Relational Operator2 : RelationalOperator  Operator=>  OutDataTypeStr=boolean  RndMeth=Simplest
  BSPR_bUCellNplErrDet_A : Outport
  BSPR_bUCellNplErrHeal_A : Outport  Port=2
  BSPR_bUCellNplErrStt_A : Outport  Port=3
  BSPR_cntUCellNplErrDet_A : Outport  Port=4
  BSPR_cntUCellNplErrHeal_A : Outport  Port=5
  BSPR_bUCellNplErrDet_flg : Outport  Port=6
  BSPR_bUCellNplErrHeal_flg : Outport  Port=7
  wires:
  BSER_rSoh/1 -> BSPR_uCellVoltNplDiag_CUR/1
  BSPR_uCellVoltNplDiag_CUR/1 -> Relational Operator1/2, Relational Operator/2, NplDiagCalc/3(BSPR_uCellVoltNplDiag_CUR)
  BSPR_uCellVolt_A/1 -> NplDiagCalc/2(BSPR_uCellVolt_A)
  BSPR_cntCellSerNum/1 -> NplDiagCalc/5(BSPR_cntCellSerNum)
  BSPR_uCellVoltMeanCoord/1 -> Add/2, Add1/1, NplDiagCalc/1(BSPR_uCellVoltMeanCoord)
  Constant1/1 -> NplDiagCalc/6(BSPR_cntUCellNplOkThres_C)
  Constant2/1 -> NplDiagCalc/7(BSPR_cntUCellNplErrThres_C)
  NplDiagCalc/3(BSPR_bUCellNplErrStt_A) -> BSPR_bUCellNplErrStt_A/1
  NplDiagCalc/4(BSPR_cntUCellNplErrDet_A) -> BSPR_cntUCellNplErrDet_A/1
  NplDiagCalc/5(BSPR_cntUCellNplErrHeal_A) -> BSPR_cntUCellNplErrHeal_A/1
  BSPR_flgCellVoltDiagEn/1 -> Logical Operator/1, NplDiagCalc/4(BSPR_flgCellVoltDiagEn)
  Constant22/1 -> CellVoltBMSDebounceStartZero8/5
  Constant21/1 -> CellVoltBMSDebounceStartZero8/3
  Constant4/1 -> CellVoltBMSDebounceStartZero8/2
  Constant3/1 -> CellVoltBMSDebounceStartZero8/4
  BSPR_uCellVoltMax/1 -> Add/1
  BSPR_uCellVoltMin/1 -> Relational Operator2/1, Add1/2
  Add/1 -> Relational Operator/1
  Add1/1 -> Relational Operator1/1
  Relational Operator/1 -> Logical Operator1/1
  Relational Operator1/1 -> Logical Operator1/2
  Logical Operator1/1 -> Logical Operator/2
  Logical Operator/1 -> CellVoltBMSDebounceStartZero8/1
  CellVoltBMSDebounceStartZero8/1 -> Logical Operator2/1, BSPR_bUCellNplErrDet_flg/1
  NplDiagCalc/1(BSPR_bUCellNplErrDet_A) -> BSPR_bUCellNplErrDet_A/1
  NplDiagCalc/2(BSPR_bUCellNplErrHeal_A) -> BSPR_bUCellNplErrHeal_A/1
  Logical Operator2/1 -> BSPR_bUCellNplErrHeal_flg/1
  Constant5/1 -> Relational Operator2/2
  Relational Operator2/1 -> Logical Operator/3

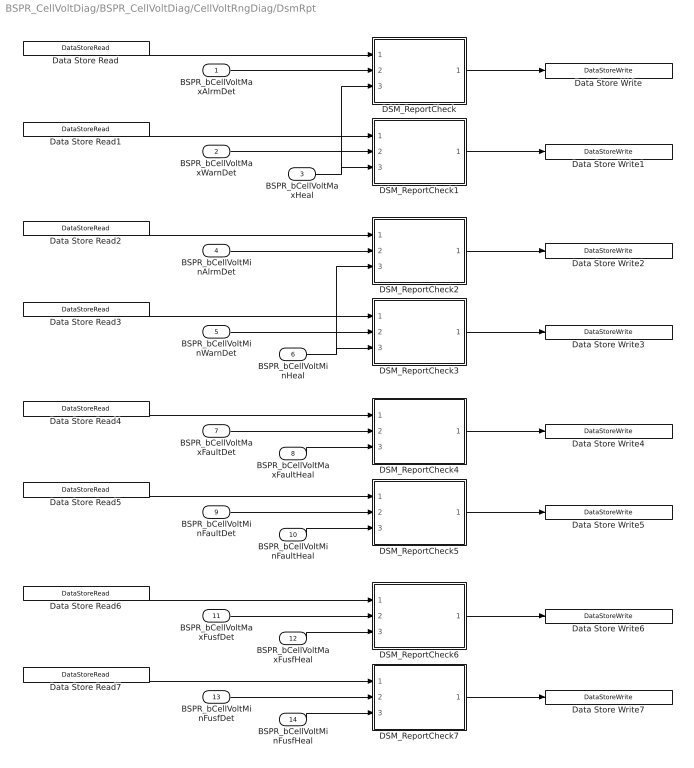
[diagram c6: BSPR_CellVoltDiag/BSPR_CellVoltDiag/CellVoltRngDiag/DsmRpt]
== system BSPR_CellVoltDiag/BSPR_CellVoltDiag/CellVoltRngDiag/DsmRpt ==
  BSPR_bCellVoltMaxAlrmDet : Inport
  BSPR_bCellVoltMaxWarnDet : Inport  Port=2
  BSPR_bCellVoltMaxHeal : Inport  Port=3
  BSPR_bCellVoltMinAlrmDet : Inport  Port=4
  BSPR_bCellVoltMinWarnDet : Inport  Port=5
  BSPR_bCellVoltMinHeal : Inport  Port=6
  BSPR_bCellVoltMaxFaultDet : Inport  Port=7
  BSPR_bCellVoltMaxFaultHeal : Inport  Port=8
  BSPR_bCellVoltMinFaultDet : Inport  Port=9
  BSPR_bCellVoltMinFaultHeal : Inport  Port=10
  BSPR_bCellVoltMaxFusfDet : Inport  Port=11
  BSPR_bCellVoltMaxFusfHeal : Inport  Port=12
  BSPR_bCellVoltMinFusfDet : Inport  Port=13
  BSPR_bCellVoltMinFusfHeal : Inport  Port=14
  DSM_ReportCheck : Subsystem  TreatAsAtomicUnit=on  RTWFcnName=DSM_ReportCheck  RTWFileName=SrvLib
  DSM_ReportCheck1 : Subsystem  TreatAsAtomicUnit=on  RTWFcnName=DSM_ReportCheck  RTWFileName=SrvLib
  DSM_ReportCheck2 : Subsystem  TreatAsAtomicUnit=on  RTWFcnName=DSM_ReportCheck  RTWFileName=SrvLib
  DSM_ReportCheck3 : Subsystem  TreatAsAtomicUnit=on  RTWFcnName=DSM_ReportCheck  RTWFileName=SrvLib
  DSM_ReportCheck4 : Subsystem  TreatAsAtomicUnit=on  RTWFcnName=DSM_ReportCheck  RTWFileName=SrvLib
  DSM_ReportCheck5 : Subsystem  TreatAsAtomicUnit=on  RTWFcnName=DSM_ReportCheck  RTWFileName=SrvLib
  DSM_ReportCheck6 : Subsystem  TreatAsAtomicUnit=on  RTWFcnName=DSM_ReportCheck  RTWFileName=SrvLib
  DSM_ReportCheck7 : Subsystem  TreatAsAtomicUnit=on  RTWFcnName=DSM_ReportCheck  RTWFileName=SrvLib
  Data Store Read : DataStoreRead  DataStoreName=DFC_CellVoltAlrmMax
  Data Store Read1 : DataStoreRead  DataStoreName=DFC_CellVoltWarnMax
  Data Store Read2 : DataStoreRead  DataStoreName=DFC_CellVoltAlrmMin
  Data Store Read3 : DataStoreRead  DataStoreName=DFC_CellVoltWarnMin
  Data Store Read4 : DataStoreRead  DataStoreName=DFC_CellVoltFaultMax
  Data Store Read5 : DataStoreRead  DataStoreName=DFC_CellVoltFaultMin
  Data Store Read6 : DataStoreRead  DataStoreName=DFC_CellVoltFusfMax
  Data Store Read7 : DataStoreRead  DataStoreName=DFC_CellVoltFusfMin
  Data Store Write : DataStoreWrite  DataStoreName=DFC_CellVoltAlrmMax
  Data Store Write1 : DataStoreWrite  DataStoreName=DFC_CellVoltWarnMax
  Data Store Write2 : DataStoreWrite  DataStoreName=DFC_CellVoltAlrmMin
  Data Store Write3 : DataStoreWrite  DataStoreName=DFC_CellVoltWarnMin
  Data Store Write4 : DataStoreWrite  DataStoreName=DFC_CellVoltFaultMax
  Data Store Write5 : DataStoreWrite  DataStoreName=DFC_CellVoltFaultMin
  Data Store Write6 : DataStoreWrite  DataStoreName=DFC_CellVoltFusfMax
  Data Store Write7 : DataStoreWrite  DataStoreName=DFC_CellVoltFusfMin
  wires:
  DSM_ReportCheck/1(Dfc_id) -> Data Store Write/1
  BSPR_bCellVoltMaxAlrmDet/1 -> DSM_ReportCheck/2(Err)
  Data Store Read/1 -> DSM_ReportCheck/1(Dfc_id_nv)
  DSM_ReportCheck2/1(Dfc_id) -> Data Store Write2/1
  BSPR_bCellVoltMinAlrmDet/1 -> DSM_ReportCheck2/2(Err)
  Data Store Read2/1 -> DSM_ReportCheck2/1(Dfc_id_nv)
  BSPR_bCellVoltMaxHeal/1 -> DSM_ReportCheck1/3(Heal), DSM_ReportCheck/3(Heal)
  DSM_ReportCheck1/1(Dfc_id) -> Data Store Write1/1
  BSPR_bCellVoltMinHeal/1 -> DSM_ReportCheck3/3(Heal), DSM_ReportCheck2/3(Heal)
  BSPR_bCellVoltMaxWarnDet/1 -> DSM_ReportCheck1/2(Err)
  Data Store Read1/1 -> DSM_ReportCheck1/1(Dfc_id_nv)
  BSPR_bCellVoltMinWarnDet/1 -> DSM_ReportCheck3/2(Err)
  Data Store Read3/1 -> DSM_ReportCheck3/1(Dfc_id_nv)
  DSM_ReportCheck3/1(Dfc_id) -> Data Store Write3/1
  BSPR_bCellVoltMaxFaultDet/1 -> DSM_ReportCheck4/2(Err)
  BSPR_bCellVoltMaxFaultHeal/1 -> DSM_ReportCheck4/3(Heal)
  BSPR_bCellVoltMinFaultDet/1 -> DSM_ReportCheck5/2(Err)
  BSPR_bCellVoltMinFaultHeal/1 -> DSM_ReportCheck5/3(Heal)
  BSPR_bCellVoltMaxFusfDet/1 -> DSM_ReportCheck6/2(Err)
  BSPR_bCellVoltMaxFusfHeal/1 -> DSM_ReportCheck6/3(Heal)
  BSPR_bCellVoltMinFusfHeal/1 -> DSM_ReportCheck7/3(Heal)
  BSPR_bCellVoltMinFusfDet/1 -> DSM_ReportCheck7/2(Err)
  Data Store Read4/1 -> DSM_ReportCheck4/1(Dfc_id_nv)
  Data Store Read5/1 -> DSM_ReportCheck5/1(Dfc_id_nv)
  Data Store Read6/1 -> DSM_ReportCheck6/1(Dfc_id_nv)
  Data Store Read7/1 -> DSM_ReportCheck7/1(Dfc_id_nv)
  DSM_ReportCheck4/1(Dfc_id) -> Data Store Write4/1
  DSM_ReportCheck5/1(Dfc_id) -> Data Store Write5/1
  DSM_ReportCheck6/1(Dfc_id) -> Data Store Write6/1
  DSM_ReportCheck7/1(Dfc_id) -> Data Store Write7/1

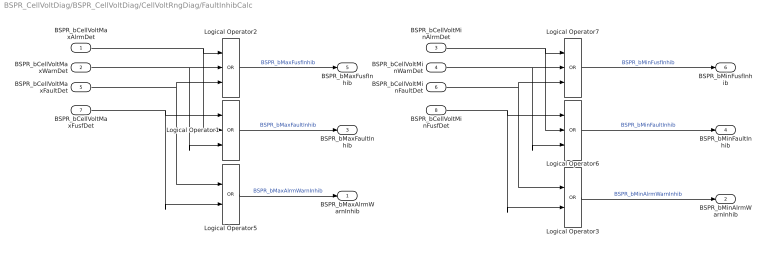
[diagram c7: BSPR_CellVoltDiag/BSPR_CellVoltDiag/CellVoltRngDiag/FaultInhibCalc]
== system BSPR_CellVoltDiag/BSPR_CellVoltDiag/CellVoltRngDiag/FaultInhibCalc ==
  BSPR_bCellVoltMaxAlrmDet : Inport
  BSPR_bCellVoltMaxWarnDet : Inport  Port=2
  BSPR_bCellVoltMinAlrmDet : Inport  Port=3
  BSPR_bCellVoltMinWarnDet : Inport  Port=4
  BSPR_bCellVoltMaxFaultDet : Inport  Port=5
  BSPR_bCellVoltMinFaultDet : Inport  Port=6
  BSPR_bCellVoltMaxFusfDet : Inport  Port=7
  BSPR_bCellVoltMinFusfDet : Inport  Port=8
  Logical Operator{1..2,6..7} (4 alike) : Logic  Operator=OR  Inputs=3  AllPortsSameDT=off  OutDataTypeStr=boolean
  Logical Operator3 : Logic  Operator=OR  AllPortsSameDT=off  OutDataTypeStr=boolean
  Logical Operator5 : Logic  Operator=OR  AllPortsSameDT=off  OutDataTypeStr=boolean
  BSPR_bMaxAlrmWarnInhib : Outport
  BSPR_bMinAlrmWarnInhib : Outport  Port=2
  BSPR_bMaxFaultInhib : Outport  Port=3
  BSPR_bMinFaultInhib : Outport  Port=4
  BSPR_bMaxFusfInhib : Outport  Port=5
  BSPR_bMinFusfInhib : Outport  Port=6
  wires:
  BSPR_bCellVoltMaxWarnDet/1 -> Logical Operator1/3, Logical Operator2/2
  BSPR_bCellVoltMaxAlrmDet/1 -> Logical Operator1/2, Logical Operator2/1
  BSPR_bCellVoltMaxFaultDet/1 -> Logical Operator5/1, Logical Operator2/3
  BSPR_bCellVoltMaxFusfDet/1 -> Logical Operator5/2, Logical Operator1/1
  BSPR_bCellVoltMinWarnDet/1 -> Logical Operator7/2, Logical Operator6/3
  BSPR_bCellVoltMinAlrmDet/1 -> Logical Operator7/1, Logical Operator6/2
  BSPR_bCellVoltMinFaultDet/1 -> Logical Operator7/3, Logical Operator3/1
  BSPR_bCellVoltMinFusfDet/1 -> Logical Operator6/1, Logical Operator3/2
  Logical Operator2/1 -> BSPR_bMaxFusfInhib/1  "BSPR_bMaxFusfInhib"
  Logical Operator1/1 -> BSPR_bMaxFaultInhib/1  "BSPR_bMaxFaultInhib"
  Logical Operator5/1 -> BSPR_bMaxAlrmWarnInhib/1  "BSPR_bMaxAlrmWarnInhib"
  Logical Operator7/1 -> BSPR_bMinFusfInhib/1  "BSPR_bMinFusfInhib"
  Logical Operator6/1 -> BSPR_bMinFaultInhib/1  "BSPR_bMinFaultInhib"
  Logical Operator3/1 -> BSPR_bMinAlrmWarnInhib/1  "BSPR_bMinAlrmWarnInhib"

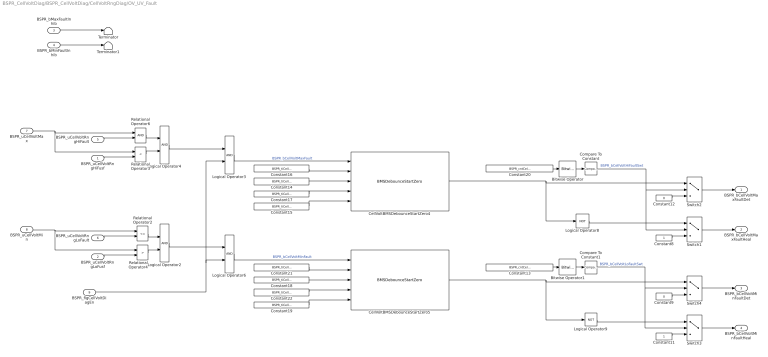
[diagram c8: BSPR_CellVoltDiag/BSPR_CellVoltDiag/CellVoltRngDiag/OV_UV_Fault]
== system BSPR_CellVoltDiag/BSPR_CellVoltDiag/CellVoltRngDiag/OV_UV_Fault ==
  BSPR_uCellVoltRngHiFusf : Inport
  BSPR_uCellVoltRngLoFusf : Inport  Port=2
  BSPR_bMaxFaultInhib : Inport  Port=3
  BSPR_bMinFaultInhib : Inport  Port=4
  BSPR_uCellVoltRngHiFault : Inport  Port=5
  BSPR_uCellVoltRngLoFault : Inport  Port=6
  BSPR_uCellVoltMax : Inport  Port=7
  BSPR_uCellVoltMin : Inport  Port=8
  BSPR_flgCellVoltDiagEn : Inport  Port=9
  Bitwise Operator : simulink/Logic and Bit Operations/Bitwise Operator  logicop=AND  UseBitMask=on  BitMask=bin2dec('00000100')  BitMaskRealWorld=Stored Integer
  Bitwise Operator1 : simulink/Logic and Bit Operations/Bitwise Operator  logicop=AND  UseBitMask=on  BitMask=bin2dec('00001000')  BitMaskRealWorld=Stored Integer
  CellVoltBMSDebounceStartZero4 : AIWAYS_Powertrain_BMS_lib/Debounce & Delay/BMSDebounceStartZero
  CellVoltBMSDebounceStartZero5 : AIWAYS_Powertrain_BMS_lib/Debounce & Delay/BMSDebounceStartZero
  Compare To Constant : simulink/Logic and Bit Operations/Compare To Constant  relop===  const=4  OutDataTypeStr=boolean
  Compare To Constant1 : simulink/Logic and Bit Operations/Compare To Constant  relop===  const=8  OutDataTypeStr=boolean
  Constant11 : Constant  OutDataTypeStr=boolean
  Constant12 : Constant  Value=0  OutDataTypeStr=boolean
  Constant13 : Constant  Value=BSPR_cntCellVoltRngDiag_CW
  Constant{14..15,18..19} (4 alike) : Constant  Value=BSPR_tiCellVoltDiagTask_C
  Constant{16..17,21..22} (4 alike) : Constant  Value=BSPR_tiCellVoltFault_C
  Constant20 : Constant  Value=BSPR_cntCellVoltRngDiag_CW
  Constant8 : Constant  OutDataTypeStr=boolean
  Constant9 : Constant  Value=0  OutDataTypeStr=boolean
  Logical Operator{2..4,6} (4 alike) : Logic  AllPortsSameDT=off  OutDataTypeStr=boolean
  Logical Operator8 : Logic  Operator=NOT  AllPortsSameDT=off  OutDataTypeStr=boolean
  Logical Operator9 : Logic  Operator=NOT  AllPortsSameDT=off  OutDataTypeStr=boolean
  Relational Operator2 : RelationalOperator  Operator=<=  OutDataTypeStr=boolean  RndMeth=Simplest
  Relational Operator3 : RelationalOperator  Operator=<  OutDataTypeStr=boolean  RndMeth=Simplest
  Relational Operator4 : RelationalOperator  Operator=>  OutDataTypeStr=boolean  RndMeth=Simplest
  Relational Operator6 : RelationalOperator  OutDataTypeStr=boolean  RndMeth=Simplest
  Switch{1..4} (4 alike) : Switch  Criteria=u2 > Threshold
  Terminator : Terminator
  Terminator1 : Terminator
  BSPR_bCellVoltMaxFaultDet : Outport
  BSPR_bCellVoltMaxFaultHeal : Outport  Port=2
  BSPR_bCellVoltMinFaultDet : Outport  Port=3
  BSPR_bCellVoltMinFaultHeal : Outport  Port=4
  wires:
  BSPR_bMinFaultInhib/1 -> Terminator1/1
  BSPR_bMaxFaultInhib/1 -> Terminator/1
  BSPR_uCellVoltMax/1 -> Relational Operator3/1, Relational Operator6/1
  BSPR_uCellVoltRngHiFault/1 -> Relational Operator6/2
  BSPR_uCellVoltRngLoFault/1 -> Relational Operator2/2
  BSPR_uCellVoltMin/1 -> Relational Operator2/1, Relational Operator4/1
  BSPR_uCellVoltRngHiFusf/1 -> Relational Operator3/2
  Relational Operator6/1 -> Logical Operator4/1
  Relational Operator3/1 -> Logical Operator4/2
  Relational Operator4/1 -> Logical Operator2/2
  Relational Operator2/1 -> Logical Operator2/1
  BSPR_uCellVoltRngLoFusf/1 -> Relational Operator4/2
  Compare To Constant/1 -> Switch1/2, Switch2/2  "BSPR_bCellVoltHiFaultSwt"
  Constant20/1 -> Bitwise Operator/1
  Bitwise Operator/1 -> Compare To Constant/1
  Switch2/1 -> BSPR_bCellVoltMaxFaultDet/1
  Constant12/1 -> Switch2/3
  Switch1/1 -> BSPR_bCellVoltMaxFaultHeal/1
  Constant8/1 -> Switch1/3
  Constant9/1 -> Switch4/3
  Constant11/1 -> Switch3/3
  Switch4/1 -> BSPR_bCellVoltMinFaultDet/1
  Switch3/1 -> BSPR_bCellVoltMinFaultHeal/1
  Constant13/1 -> Bitwise Operator1/1
  Bitwise Operator1/1 -> Compare To Constant1/1
  Compare To Constant1/1 -> Switch3/2, Switch4/2  "BSPR_bCellVoltLoFaultSwt"
  Logical Operator4/1 -> Logical Operator3/1
  Logical Operator2/1 -> Logical Operator6/1
  BSPR_flgCellVoltDiagEn/1 -> Logical Operator3/2, Logical Operator6/2
  Constant17/1 -> CellVoltBMSDebounceStartZero4/4
  Constant15/1 -> CellVoltBMSDebounceStartZero4/5
  Constant14/1 -> CellVoltBMSDebounceStartZero4/3
  Constant16/1 -> CellVoltBMSDebounceStartZero4/2
  Constant21/1 -> CellVoltBMSDebounceStartZero5/2
  Constant18/1 -> CellVoltBMSDebounceStartZero5/3
  Constant19/1 -> CellVoltBMSDebounceStartZero5/5
  Constant22/1 -> CellVoltBMSDebounceStartZero5/4
  Logical Operator6/1 -> CellVoltBMSDebounceStartZero5/1  "BSPR_bCellVoltMinFault"
  Logical Operator3/1 -> CellVoltBMSDebounceStartZero4/1  "BSPR_bCellVoltMaxFault"
  CellVoltBMSDebounceStartZero4/1 -> Logical Operator8/1, Switch2/1
  CellVoltBMSDebounceStartZero5/1 -> Logical Operator9/1, Switch4/1
  Logical Operator8/1 -> Switch1/1
  Logical Operator9/1 -> Switch3/1

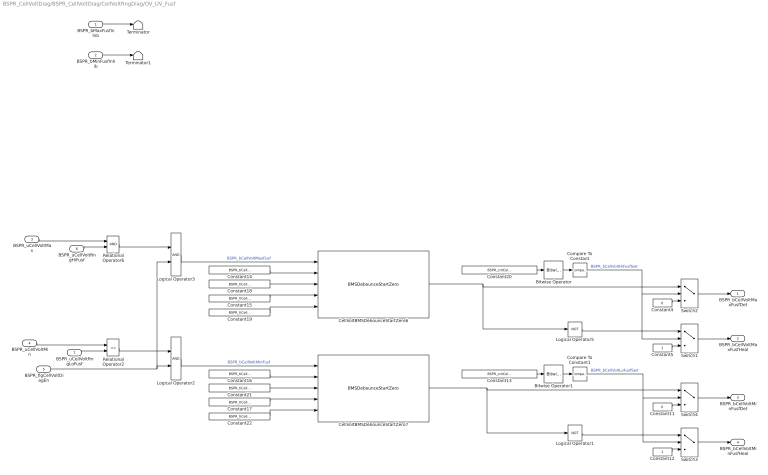
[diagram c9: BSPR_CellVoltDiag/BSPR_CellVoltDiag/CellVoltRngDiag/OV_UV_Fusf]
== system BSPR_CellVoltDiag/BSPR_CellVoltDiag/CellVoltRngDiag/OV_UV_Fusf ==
  BSPR_bMaxFusfInhib : Inport
  BSPR_bMinFusfInhib : Inport  Port=2
  BSPR_uCellVoltMax : Inport  Port=3
  BSPR_uCellVoltMin : Inport  Port=4
  BSPR_flgCellVoltDiagEn : Inport  Port=5
  BSPR_uCellVoltRngHiFusf : Inport  Port=6
  BSPR_uCellVoltRngLoFusf : Inport  Port=7
  Bitwise Operator : simulink/Logic and Bit Operations/Bitwise Operator  logicop=AND  UseBitMask=on  BitMask=bin2dec('00010000')  BitMaskRealWorld=Stored Integer
  Bitwise Operator1 : simulink/Logic and Bit Operations/Bitwise Operator  logicop=AND  UseBitMask=on  BitMask=bin2dec('00100000')  BitMaskRealWorld=Stored Integer
  CellVoltBMSDebounceStartZero6 : AIWAYS_Powertrain_BMS_lib/Debounce & Delay/BMSDebounceStartZero
  CellVoltBMSDebounceStartZero7 : AIWAYS_Powertrain_BMS_lib/Debounce & Delay/BMSDebounceStartZero
  Compare To Constant : simulink/Logic and Bit Operations/Compare To Constant  relop===  const=16  OutDataTypeStr=boolean
  Compare To Constant1 : simulink/Logic and Bit Operations/Compare To Constant  relop===  const=32  OutDataTypeStr=boolean
  Constant11 : Constant  Value=0  OutDataTypeStr=boolean
  Constant12 : Constant  OutDataTypeStr=boolean
  Constant13 : Constant  Value=BSPR_cntCellVoltRngDiag_CW
  Constant{14..17} (4 alike) : Constant  Value=BSPR_tiCellVoltFusf_C
  Constant{18..19,21..22} (4 alike) : Constant  Value=BSPR_tiCellVoltDiagTask_C
  Constant20 : Constant  Value=BSPR_cntCellVoltRngDiag_CW
  Constant4 : Constant  Value=0  OutDataTypeStr=boolean
  Constant5 : Constant  OutDataTypeStr=boolean
  Logical Operator1 : Logic  Operator=NOT  AllPortsSameDT=off  OutDataTypeStr=boolean
  Logical Operator2 : Logic  AllPortsSameDT=off  OutDataTypeStr=boolean
  Logical Operator3 : Logic  AllPortsSameDT=off  OutDataTypeStr=boolean
  Logical Operator5 : Logic  Operator=NOT  AllPortsSameDT=off  OutDataTypeStr=boolean
  Relational Operator2 : RelationalOperator  Operator=<=  OutDataTypeStr=boolean  RndMeth=Simplest
  Relational Operator6 : RelationalOperator  OutDataTypeStr=boolean  RndMeth=Simplest
  Switch{1..4} (4 alike) : Switch  Criteria=u2 > Threshold
  Terminator : Terminator
  Terminator1 : Terminator
  BSPR_bCellVoltMaxFusfDet : Outport
  BSPR_bCellVoltMaxFusfHeal : Outport  Port=2
  BSPR_bCellVoltMinFusfDet : Outport  Port=3
  BSPR_bCellVoltMinFusfHeal : Outport  Port=4
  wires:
  BSPR_uCellVoltRngLoFusf/1 -> Relational Operator2/2
  BSPR_uCellVoltMin/1 -> Relational Operator2/1
  BSPR_uCellVoltRngHiFusf/1 -> Relational Operator6/2
  BSPR_uCellVoltMax/1 -> Relational Operator6/1
  BSPR_bMaxFusfInhib/1 -> Terminator/1
  BSPR_bMinFusfInhib/1 -> Terminator1/1
  Compare To Constant/1 -> Switch1/2, Switch2/2  "BSPR_bCellVoltHiFusfSwt"
  Constant20/1 -> Bitwise Operator/1
  Bitwise Operator/1 -> Compare To Constant/1
  Constant4/1 -> Switch2/3
  Switch2/1 -> BSPR_bCellVoltMaxFusfDet/1
  Constant5/1 -> Switch1/3
  Switch1/1 -> BSPR_bCellVoltMaxFusfHeal/1
  CellVoltBMSDebounceStartZero6/1 -> Logical Operator5/1, Switch2/1
  Relational Operator6/1 -> Logical Operator3/1
  Relational Operator2/1 -> Logical Operator2/1
  BSPR_flgCellVoltDiagEn/1 -> Logical Operator3/2, Logical Operator2/2
  Compare To Constant1/1 -> Switch3/2, Switch4/2  "BSPR_bCellVoltLoFusfSwt"
  Constant11/1 -> Switch4/3
  Constant12/1 -> Switch3/3
  CellVoltBMSDebounceStartZero7/1 -> Logical Operator1/1, Switch4/1
  Switch4/1 -> BSPR_bCellVoltMinFusfDet/1
  Switch3/1 -> BSPR_bCellVoltMinFusfHeal/1
  Constant13/1 -> Bitwise Operator1/1
  Bitwise Operator1/1 -> Compare To Constant1/1
  Constant19/1 -> CellVoltBMSDebounceStartZero6/5
  Constant18/1 -> CellVoltBMSDebounceStartZero6/3
  Constant15/1 -> CellVoltBMSDebounceStartZero6/4
  Constant14/1 -> CellVoltBMSDebounceStartZero6/2
  Constant22/1 -> CellVoltBMSDebounceStartZero7/5
  Constant21/1 -> CellVoltBMSDebounceStartZero7/3
  Constant16/1 -> CellVoltBMSDebounceStartZero7/2
  Constant17/1 -> CellVoltBMSDebounceStartZero7/4
  Logical Operator3/1 -> CellVoltBMSDebounceStartZero6/1  "BSPR_bCellVoltMaxFusf"
  Logical Operator5/1 -> Switch1/1
  Logical Operator2/1 -> CellVoltBMSDebounceStartZero7/1  "BSPR_bCellVoltMinFusf"
  Logical Operator1/1 -> Switch3/1
